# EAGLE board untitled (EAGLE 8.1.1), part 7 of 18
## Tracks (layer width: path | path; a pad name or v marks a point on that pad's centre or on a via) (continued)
S$6634 (continued)
  Bottom 0: 111.83,160.68 111.78,160.73
S$6635
  Bottom 0: 111.78,160.73 111.71,160.77
S$6636
  Bottom 0: 111.71,160.77 111.63,160.78
S$6637
  Bottom 0: 111.63,160.78 111.19,160.78
S$6638
  Bottom 0: 111.19,160.78 111.19,160.91
S$6639
  Bottom 0: 111.19,160.91 111.12,161.13
S$6640
  Bottom 0: 111.12,161.13 110.96,161.29
S$6641
  Bottom 0: 110.96,161.29 110.74,161.35
S$6642
  Bottom 0: 110.74,161.35 110.39,161.35
S$6643
  Bottom 0: 110.39,161.35 109.3,162.43
S$6644
  Bottom 0: 109.3,162.43 109.36,162.57
S$6645
  Bottom 0: 109.36,162.57 109.41,162.89
S$6646
  Bottom 0: 109.41,162.89 109.36,163.22
S$6647
  Bottom 0: 109.36,163.22 109.23,163.51
S$6648
  Bottom 0: 109.23,163.51 109.03,163.77
S$6649
  Bottom 0: 109.03,163.77 108.76,163.96
S$6650
  Bottom 0: 108.76,163.96 108.46,164.06
S$6651
  Bottom 0: 108.46,164.06 108.13,164.08
S$6652
  Bottom 0: 108.13,164.08 107.81,164.02
S$6653
  Bottom 0: 107.81,164.02 107.52,163.87
S$6654
  Bottom 0: 107.52,163.87 107.29,163.65
S$6655
  Bottom 0: 107.29,163.65 107.12,163.37
S$6656
  Bottom 0: 107.12,163.37 107.03,163.06
S$6657
  Bottom 0: 107.03,163.06 107.03,162.73
S$6658
  Bottom 0: 107.03,162.73 107.12,162.42
S$6659
  Bottom 0: 107.12,162.42 107.29,162.14
S$6660
  Bottom 0: 107.29,162.14 107.52,161.92
S$6661
  Bottom 0: 107.52,161.92 107.81,161.77
S$6662
  Bottom 0: 107.81,161.77 108.13,161.71
S$6663
  Bottom 0: 108.13,161.71 108.46,161.73
S$6664
  Bottom 0: 108.46,161.73 108.68,161.8
S$6665
  Bottom 0: 108.68,161.8 109.74,160.75
S$6666
  Bottom 0: 109.74,160.75 109.7,160.73
S$6667
  Bottom 0: 109.7,160.73 109.65,160.68
S$6668
  Bottom 0: 109.65,160.68 109.61,160.6
S$6669
  Bottom 0: 109.61,160.6 109.6,160.53
S$6670
  Bottom 0: 109.6,160.53 109.6,159.04
S$6671
  Bottom 0: 109.6,159.04 105.97,162.67
S$6672
  Bottom 0: 105.97,162.67 106.01,162.88
S$6673
  Bottom 0: 106.01,162.88 105.96,163.13
S$6674
  Bottom 0: 105.96,163.13 105.83,163.34
S$6675
  Bottom 0: 105.83,163.34 105.63,163.5
S$6676
  Bottom 0: 105.63,163.5 105.4,163.55
S$6677
  Bottom 0: 105.4,163.55 105.97,164.13
S$6678
  Bottom 0: 105.97,164.13 106.23,164.08
S$6679
  Bottom 0: 106.23,164.08 106.55,164.1
S$6680
  Bottom 0: 106.55,164.1 106.86,164.21
S$6681
  Bottom 0: 106.86,164.21 107.12,164.39
S$6682
  Bottom 0: 107.12,164.39 107.33,164.65
S$6683
  Bottom 0: 107.33,164.65 107.45,164.95
S$6684
  Bottom 0: 107.45,164.95 107.5,165.27
S$6685
  Bottom 0: 107.5,165.27 107.45,165.59
S$6686
  Bottom 0: 107.45,165.59 107.33,165.89
S$6687
  Bottom 0: 107.33,165.89 107.12,166.14
S$6688
  Bottom 0: 107.12,166.14 107.98,166.14
S$6689
  Bottom 0: 107.98,166.14 113.35,160.77
S$6690
  Bottom 0: 113.35,160.77 113.12,160.77
S$6691
  Bottom 0: 113.12,160.77 112.81,160.68
S$6692
  Bottom 0: 112.81,160.68 112.53,160.5
S$6693
  Bottom 0: 112.53,160.5 112.32,160.26
S$6694
  Bottom 0: 112.32,160.26 112.18,159.96
S$6695
  Bottom 0: 112.18,159.96 112.14,159.64
S$6696
  Bottom 0: 112.14,159.64 112.18,159.32
S$6697
  Bottom 0: 112.18,159.32 112.32,159.02
S$6698
  Bottom 0: 112.32,159.02 112.53,158.78
S$6699
  Bottom 0: 112.53,158.78 112.81,158.6
S$6700
  Bottom 0: 112.81,158.6 113.12,158.51
S$6701
  Bottom 0: 113.12,158.51 113.45,158.51
S$6702
  Bottom 0: 113.45,158.51 113.76,158.6
S$6703
  Bottom 0: 113.76,158.6 114.03,158.78
S$6704
  Bottom 0: 114.03,158.78 114.24,159.02
S$6705
  Bottom 0: 114.24,159.02 114.38,159.32
S$6706
  Bottom 0: 114.38,159.32 114.43,159.64
S$6707
  Bottom 0: 114.43,159.64 114.42,159.71
S$6708
  Bottom 0: 114.42,159.71 123.49,150.63
S$6709
  Bottom 0: 123.49,150.63 123.49,131.46
S$6710
  Bottom 0: 123.49,131.46 113.33,121.3
S$6711
  Bottom 0: 113.33,121.3 113.29,121.24
S$6712
  Bottom 0: 113.29,121.24 113.25,121.18
S$6713
  Bottom 0: 113.25,121.18 113.22,121.12
S$6714
  Bottom 0: 113.22,121.12 113.21,121.06
S$6715
  Bottom 0: 113.21,121.06 113.2,120.98
S$6716
  Bottom 0: 113.2,120.98 113.2,113.26
S$6717
  Bottom 0: 113.2,113.26 113.06,113.11
S$6718
  Bottom 0: 113.06,113.11 112.97,112.88
S$6719
  Bottom 0: 112.97,112.88 112.97,112.62
S$6720
  Bottom 0: 112.97,112.62 113.06,112.39
S$6721
  Bottom 0: 113.06,112.39 113.23,112.2
S$6722
  Bottom 0: 113.23,112.2 113.45,112.09
S$6723
  Bottom 0: 113.45,112.09 113.71,112.07
S$6724
  Bottom 0: 113.71,112.07 113.95,112.14
S$6725
  Bottom 0: 113.95,112.14 114.15,112.29
S$6726
  Bottom 0: 114.15,112.29 114.28,112.5
S$6727
  Bottom 0: 114.28,112.5 114.33,112.75
S$6728
  Bottom 0: 114.33,112.75 114.28,113
S$6729
  Bottom 0: 114.28,113 114.15,113.21
S$6730
  Bottom 0: 114.15,113.21 114.09,113.26
S$6731
  Bottom 0: 114.09,113.26 114.09,120.8
S$6732
  Bottom 0: 114.09,120.8 124.25,130.96
S$6733
  Bottom 0: 124.25,130.96 124.29,131.01
S$6734
  Bottom 0: 124.29,131.01 124.33,131.07
S$6735
  Bottom 0: 124.33,131.07 124.35,131.13
S$6736
  Bottom 0: 124.35,131.13 124.37,131.2
S$6737
  Bottom 0: 124.37,131.2 124.37,131.27
S$6738
  Bottom 0: 124.37,131.27 124.37,147.41
S$6739
  Bottom 0: 124.37,147.41 130.71,147.41
S$6740
  Bottom 0: 130.71,147.41 130.78,147.42
S$6741
  Bottom 0: 130.78,147.42 130.85,147.43
S$6742
  Bottom 0: 130.85,147.43 130.91,147.46
S$6743
  Bottom 0: 130.91,147.46 130.97,147.5
S$6744
  Bottom 0: 130.97,147.5 131.02,147.54
S$6745
  Bottom 0: 131.02,147.54 134.25,150.77
S$6746
  Bottom 0: 134.25,150.77 134.28,150.75
S$6747
  Bottom 0: 134.28,150.75 134.61,150.65
S$6748
  Bottom 0: 134.61,150.65 134.96,150.63
S$6749
  Bottom 0: 134.96,150.63 135.31,150.69
S$6750
  Bottom 0: 135.31,150.69 135.62,150.84
S$6751
  Bottom 0: 135.62,150.84 135.89,151.06
S$6752
  Bottom 0: 135.89,151.06 136.1,151.35
S$6753
  Bottom 0: 136.1,151.35 136.22,151.67
S$6754
  Bottom 0: 136.22,151.67 136.27,152.02
S$6755
  Bottom 0: 136.27,152.02 136.22,152.36
S$6756
  Bottom 0: 136.22,152.36 136.1,152.69
S$6757
  Bottom 0: 136.1,152.69 135.89,152.97
S$6758
  Bottom 0: 135.89,152.97 135.62,153.2
S$6759
  Bottom 0: 135.62,153.2 135.31,153.35
S$6760
  Bottom 0: 135.31,153.35 134.96,153.41
S$6761
  Bottom 0: 134.96,153.41 134.61,153.39
S$6762
  Bottom 0: 134.61,153.39 134.28,153.28
S$6763
  Bottom 0: 134.28,153.28 133.99,153.1
S$6764
  Bottom 0: 133.99,153.1 133.74,152.84
S$6765
  Bottom 0: 133.74,152.84 133.57,152.53
S$6766
  Bottom 0: 133.57,152.53 133.49,152.19
S$6767
  Bottom 0: 133.49,152.19 133.49,151.84
S$6768
  Bottom 0: 133.49,151.84 133.57,151.51
S$6769
  Bottom 0: 133.57,151.51 133.63,151.4
S$6770
  Bottom 0: 133.63,151.4 130.52,148.29
S$6771
  Bottom 0: 130.52,148.29 129.26,148.29
S$6772
  Bottom 0: 129.26,148.29 129.27,148.3
S$6773
  Bottom 0: 129.27,148.3 129.54,148.52
S$6774
  Bottom 0: 129.54,148.52 129.75,148.81
S$6775
  Bottom 0: 129.75,148.81 129.88,149.13
S$6776
  Bottom 0: 129.88,149.13 129.92,149.48
S$6777
  Bottom 0: 129.92,149.48 129.88,149.82
S$6778
  Bottom 0: 129.88,149.82 129.75,150.15
S$6779
  Bottom 0: 129.75,150.15 129.54,150.43
S$6780
  Bottom 0: 129.54,150.43 129.27,150.66
S$6781
  Bottom 0: 129.27,150.66 128.96,150.81
S$6782
  Bottom 0: 128.96,150.81 128.61,150.87
S$6783
  Bottom 0: 128.61,150.87 128.26,150.85
S$6784
  Bottom 0: 128.26,150.85 127.93,150.74
S$6785
  Bottom 0: 127.93,150.74 127.64,150.56
S$6786
  Bottom 0: 127.64,150.56 127.39,150.3
S$6787
  Bottom 0: 127.39,150.3 127.22,149.99
S$6788
  Bottom 0: 127.22,149.99 127.14,149.65
S$6789
  Bottom 0: 127.14,149.65 127.14,149.3
S$6790
  Bottom 0: 127.14,149.3 127.22,148.97
S$6791
  Bottom 0: 127.22,148.97 127.39,148.66
S$6792
  Bottom 0: 127.39,148.66 127.64,148.4
S$6793
  Bottom 0: 127.64,148.4 127.8,148.29
S$6794
  Bottom 0: 127.8,148.29 124.37,148.29
S$6795
  Bottom 0: 124.37,148.29 124.37,150.81
S$6796
  Bottom 0: 124.37,150.81 124.37,150.89
S$6797
  Bottom 0: 124.37,150.89 124.35,150.95
S$6798
  Bottom 0: 124.35,150.95 124.33,151.01
S$6799
  Bottom 0: 124.33,151.01 124.29,151.07
S$6800
  Bottom 0: 124.29,151.07 124.25,151.13
S$6801
  Bottom 0: 124.25,151.13 108.48,166.9
S$6802
  Bottom 0: 108.48,166.9 108.37,166.98
S$6803
  Bottom 0: 108.37,166.98 108.31,167
S$6804
  Bottom 0: 108.31,167 108.24,167.02
S$6805
  Bottom 0: 108.24,167.02 108.17,167.03
S$6806
  Bottom 0: 108.17,167.03 104.53,167.03
S$6807
  Bottom 0: 104.53,167.03 104.45,167.02
S$6808
  Bottom 0: 104.45,167.02 104.39,167
S$6809
  Bottom 0: 104.39,167 104.32,166.97
S$6810
  Bottom 0: 104.32,166.97 104.27,166.94
S$6811
  Bottom 0: 104.27,166.94 104.21,166.89
S$6812
  Bottom 0: 104.21,166.89 101.72,164.4
S$6813
  Bottom 0: 101.72,164.4 99.51,164.4
S$6814
  Bottom 0: 99.51,164.4 99.71,164.65
S$6815
  Bottom 0: 99.71,164.65 99.83,164.95
S$6816
  Bottom 0: 99.83,164.95 99.88,165.27
S$6817
  Bottom 0: 99.88,165.27 99.83,165.59
S$6818
  Bottom 0: 99.83,165.59 99.71,165.89
S$6819
  Bottom 0: 99.71,165.89 99.5,166.14
S$6820
  Bottom 0: 99.5,166.14 99.24,166.33
S$6821
  Bottom 0: 99.24,166.33 98.93,166.44
S$6822
  Bottom 0: 98.93,166.44 98.63,166.46
S$6823
  Bottom 0: 98.63,166.46 98.63,168.08
S$6824
  Bottom 0: 98.63,168.08 98.65,168.02
S$6825
  Bottom 0: 98.65,168.02 98.82,167.71
S$6826
  Bottom 0: 98.82,167.71 99.06,167.45
S$6827
  Bottom 0: 99.06,167.45 99.36,167.26
S$6828
  Bottom 0: 99.36,167.26 99.69,167.16
S$6829
  Bottom 0: 99.69,167.16 100.03,167.14
S$6830
  Bottom 0: 100.03,167.14 100.38,167.2
S$6831
  Bottom 0: 100.38,167.2 100.7,167.35
S$6832
  Bottom 0: 100.7,167.35 100.97,167.57
S$6833
  Bottom 0: 100.97,167.57 101.17,167.86
S$6834
  Bottom 0: 101.17,167.86 101.3,168.18
S$6835
  Bottom 0: 101.3,168.18 101.35,168.53
S$6836
  Bottom 0: 101.35,168.53 101.3,168.87
S$6837
  Bottom 0: 101.3,168.87 101.17,169.2
S$6838
  Bottom 0: 101.17,169.2 100.97,169.48
S$6839
  Bottom 0: 100.97,169.48 100.7,169.71
S$6840
  Bottom 0: 100.7,169.71 100.38,169.86
S$6841
  Bottom 0: 100.38,169.86 100.03,169.92
S$6842
  Bottom 0: 100.03,169.92 99.69,169.9
S$6843
  Bottom 0: 99.69,169.9 99.36,169.79
S$6844
  Bottom 0: 99.36,169.79 99.06,169.61
S$6845
  Bottom 0: 99.06,169.61 98.82,169.35
S$6846
  Bottom 0: 98.82,169.35 98.65,169.04
S$6847
  Bottom 0: 98.65,169.04 98.63,168.99
S$6848
  Bottom 0: 98.63,168.99 98.63,174.21
S$6849
  Bottom 0: 98.63,174.21 101.53,177.1
S$6850
  Bottom 0: 101.53,177.1 101.56,177.16
S$6851
  Bottom 0: 101.56,177.16 101.6,177.2
S$6852
  Bottom 0: 101.6,177.2 101.61,177.25
S$6853
  Bottom 0: 101.61,177.25 101.64,177.3
S$6854
  Bottom 0: 101.64,177.3 101.64,177.36
S$6855
  Bottom 0: 101.64,177.36 101.66,177.42
S$6856
  Bottom 0: 101.66,177.42 101.66,177.55
S$6857
  Bottom 0: 101.66,177.55 102.11,177.55
S$6858
  Bottom 0: 102.11,177.55 102.18,177.56
S$6859
  Bottom 0: 102.18,177.56 102.25,177.6
S$6860
  Bottom 0: 102.25,177.6 102.31,177.65
S$6861
  Bottom 0: 102.31,177.65 102.35,177.72
S$6862
  Bottom 0: 102.35,177.72 102.36,177.8
S$6863
  Bottom 0: 102.36,177.8 102.36,179.51
S$6864
  Bottom 0: 102.36,179.51 102.97,179.51
S$6865
  Bottom 0: 102.97,179.51 102.8,179.31
S$6866
  Bottom 0: 102.8,179.31 102.66,179.01
S$6867
  Bottom 0: 102.66,179.01 102.62,178.69
S$6868
  Bottom 0: 102.62,178.69 102.66,178.37
S$6869
  Bottom 0: 102.66,178.37 102.8,178.07
S$6870
  Bottom 0: 102.8,178.07 103.01,177.82
S$6871
  Bottom 0: 103.01,177.82 103.29,177.65
S$6872
  Bottom 0: 103.29,177.65 103.6,177.56
S$6873
  Bottom 0: 103.6,177.56 103.92,177.56
S$6874
  Bottom 0: 103.92,177.56 104.23,177.65
S$6875
  Bottom 0: 104.23,177.65 104.51,177.82
S$6876
  Bottom 0: 104.51,177.82 104.72,178.07
S$6877
  Bottom 0: 104.72,178.07 104.86,178.37
S$6878
  Bottom 0: 104.86,178.37 104.9,178.69
S$6879
  Bottom 0: 104.9,178.69 104.86,179.01
S$6880
  Bottom 0: 104.86,179.01 104.72,179.31
S$6881
  Bottom 0: 104.72,179.31 104.55,179.51
S$6882
  Bottom 0: 104.55,179.51 119.13,179.51
S$6883
  Bottom 0: 119.13,179.51 119.13,177.8
S$6884
  Bottom 0: 119.13,177.8 119.14,177.72
S$6885
  Bottom 0: 119.14,177.72 119.18,177.65
S$6886
  Bottom 0: 119.18,177.65 119.23,177.6
S$6887
  Bottom 0: 119.23,177.6 119.3,177.56
S$6888
  Bottom 0: 119.3,177.56 119.38,177.55
S$6889
  Bottom 0: 119.38,177.55 119.77,177.55
S$6890
  Bottom 0: 119.77,177.55 117.11,174.89
S$6891
  Bottom 0: 117.11,174.89 117.07,174.84
S$6892
  Bottom 0: 117.07,174.84 117.03,174.78
S$6893
  Bottom 0: 117.03,174.78 117,174.72
S$6894
  Bottom 0: 117,174.72 116.99,174.65
S$6895
  Bottom 0: 116.99,174.65 116.98,174.58
S$6896
  Bottom 0: 116.98,174.58 116.98,166.19
S$6897
  Bottom 0: 116.98,166.19 116.81,166.03
S$6898
  Bottom 0: 116.81,166.03 116.64,165.75
S$6899
  Bottom 0: 116.64,165.75 116.56,165.43
S$6900
  Bottom 0: 116.56,165.43 116.56,165.11
S$6901
  Bottom 0: 116.56,165.11 116.64,164.79
S$6902
  Bottom 0: 116.64,164.79 116.71,164.68
S$6903
  Bottom 0: 116.71,164.68 113.93,167.46
S$6904
  Bottom 0: 113.93,167.46 113.88,167.5
S$6905
  Bottom 0: 113.88,167.5 113.82,167.54
S$6906
  Bottom 0: 113.82,167.54 113.76,167.56
S$6907
  Bottom 0: 113.76,167.56 113.69,167.58
S$6908
  Bottom 0: 113.69,167.58 113.62,167.58
S$6909
  Bottom 0: 113.62,167.58 110.41,167.58
S$6910
  Bottom 0: 110.41,167.58 107.54,170.45
S$6911
  Bottom 0: 107.54,170.45 107.65,170.72
S$6912
  Bottom 0: 107.65,170.72 107.7,171.07
S$6913
  Bottom 0: 107.7,171.07 107.65,171.41
S$6914
  Bottom 0: 107.65,171.41 107.52,171.74
S$6915
  Bottom 0: 107.52,171.74 107.31,172.02
S$6916
  Bottom 0: 107.31,172.02 107.05,172.25
S$6917
  Bottom 0: 107.05,172.25 106.73,172.4
S$6918
  Bottom 0: 106.73,172.4 106.39,172.46
S$6919
  Bottom 0: 106.39,172.46 106.03,172.44
S$6920
  Bottom 0: 106.03,172.44 105.7,172.33
S$6921
  Bottom 0: 105.7,172.33 105.41,172.15
S$6922
  Bottom 0: 105.41,172.15 105.17,171.89
S$6923
  Bottom 0: 105.17,171.89 105,171.58
S$6924
  Bottom 0: 105,171.58 104.91,171.24
S$6925
  Bottom 0: 104.91,171.24 104.91,170.9
S$6926
  Bottom 0: 104.91,170.9 105,170.56
S$6927
  Bottom 0: 105,170.56 105.17,170.25
S$6928
  Bottom 0: 105.17,170.25 105.41,169.99
S$6929
  Bottom 0: 105.41,169.99 105.7,169.8
S$6930
  Bottom 0: 105.7,169.8 106.03,169.7
S$6931
  Bottom 0: 106.03,169.7 106.39,169.68
S$6932
  Bottom 0: 106.39,169.68 106.73,169.74
S$6933
  Bottom 0: 106.73,169.74 106.91,169.82
S$6934
  Bottom 0: 106.91,169.82 109.91,166.83
S$6935
  Bottom 0: 109.91,166.83 109.97,166.79
S$6936
  Bottom 0: 109.97,166.79 110.03,166.75
S$6937
  Bottom 0: 110.03,166.75 110.09,166.72
S$6938
  Bottom 0: 110.09,166.72 110.15,166.71
S$6939
  Bottom 0: 110.15,166.71 110.23,166.7
S$6940
  Bottom 0: 110.23,166.7 113.43,166.7
S$6941
  Bottom 0: 113.43,166.7 116.07,164.06
S$6942
  Bottom 0: 116.07,164.06 115.75,164.08
S$6943
  Bottom 0: 115.75,164.08 115.43,164.02
S$6944
  Bottom 0: 115.43,164.02 115.14,163.87
S$6945
  Bottom 0: 115.14,163.87 114.91,163.65
S$6946
  Bottom 0: 114.91,163.65 114.74,163.37
S$6947
  Bottom 0: 114.74,163.37 114.65,163.06
S$6948
  Bottom 0: 114.65,163.06 114.65,162.73
S$6949
  Bottom 0: 114.65,162.73 114.74,162.42
S$6950
  Bottom 0: 114.74,162.42 114.91,162.14
S$6951
  Bottom 0: 114.91,162.14 115.14,161.92
S$6952
  Bottom 0: 115.14,161.92 115.43,161.77
S$6953
  Bottom 0: 115.43,161.77 115.75,161.71
S$6954
  Bottom 0: 115.75,161.71 116.08,161.73
S$6955
  Bottom 0: 116.08,161.73 116.38,161.83
S$6956
  Bottom 0: 116.38,161.83 116.65,162.02
S$6957
  Bottom 0: 116.65,162.02 116.85,162.28
S$6958
  Bottom 0: 116.85,162.28 116.88,162.33
S$6959
  Bottom 0: 116.88,162.33 123.05,162.33
S$6960
  Bottom 0: 123.05,162.33 123.14,162.33
S$6961
  Bottom 0: 123.14,162.33 123.23,162.35
S$6962
  Bottom 0: 123.23,162.35 123.31,162.38
S$6963
  Bottom 0: 123.31,162.38 123.38,162.43
S$6964
  Bottom 0: 123.38,162.43 123.45,162.49
S$6965
  Bottom 0: 123.45,162.49 125.08,164.12
S$6966
  Bottom 0: 125.08,164.12 125.28,164.08
S$6967
  Bottom 0: 125.28,164.08 125.6,164.1
S$6968
  Bottom 0: 125.6,164.1 125.91,164.21
S$6969
  Bottom 0: 125.91,164.21 126.17,164.4
S$6970
  Bottom 0: 126.17,164.4 126.37,164.64
S$6971
  Bottom 0: 126.37,164.64 132.34,164.64
S$6972
  Bottom 0: 132.34,164.64 133.75,163.23
S$6973
  Bottom 0: 133.75,163.23 133.71,163.06
S$6974
  Bottom 0: 133.71,163.06 133.71,162.73
S$6975
  Bottom 0: 133.71,162.73 133.79,162.42
S$6976
  Bottom 0: 133.79,162.42 133.96,162.14
S$6977
  Bottom 0: 133.96,162.14 134.2,161.92
S$6978
  Bottom 0: 134.2,161.92 134.49,161.77
S$6979
  Bottom 0: 134.49,161.77 134.81,161.71
S$6980
  Bottom 0: 134.81,161.71 135.13,161.73
S$6981
  Bottom 0: 135.13,161.73 135.44,161.83
S$6982
  Bottom 0: 135.44,161.83 135.7,162.02
S$6983
  Bottom 0: 135.7,162.02 135.91,162.28
S$6984
  Bottom 0: 135.91,162.28 136.04,162.57
S$6985
  Bottom 0: 136.04,162.57 136.08,162.89
S$6986
  Bottom 0: 136.08,162.89 136.04,163.22
S$6987
  Bottom 0: 136.04,163.22 135.96,163.39
S$6988
  Bottom 0: 135.96,163.39 145.01,163.39
S$6989
  Bottom 0: 145.01,163.39 145.08,163.4
S$6990
  Bottom 0: 145.08,163.4 145.15,163.41
S$6991
  Bottom 0: 145.15,163.41 145.2,163.44
S$6992
  Bottom 0: 145.2,163.44 145.26,163.48
S$6993
  Bottom 0: 145.26,163.48 145.31,163.51
S$6994
  Bottom 0: 145.31,163.51 145.22,163.37
S$6995
  Bottom 0: 145.22,163.37 145.14,163.06
S$6996
  Bottom 0: 145.14,163.06 145.14,162.73
S$6997
  Bottom 0: 145.14,162.73 145.22,162.42
S$6998
  Bottom 0: 145.22,162.42 145.39,162.14
S$6999
  Bottom 0: 145.39,162.14 145.63,161.92
S$7000
  Bottom 0: 145.63,161.92 145.92,161.77
S$7001
  Bottom 0: 145.92,161.77 146.24,161.71
S$7002
  Bottom 0: 146.24,161.71 146.56,161.73
S$7003
  Bottom 0: 146.56,161.73 146.78,161.8
S$7004
  Bottom 0: 146.78,161.8 147.84,160.75
S$7005
  Bottom 0: 147.84,160.75 147.81,160.73
S$7006
  Bottom 0: 147.81,160.73 147.75,160.68
S$7007
  Bottom 0: 147.75,160.68 147.71,160.6
S$7008
  Bottom 0: 147.71,160.6 147.7,160.53
S$7009
  Bottom 0: 147.7,160.53 147.7,158.75
S$7010
  Bottom 0: 147.7,158.75 147.71,158.67
S$7011
  Bottom 0: 147.71,158.67 147.75,158.6
S$7012
  Bottom 0: 147.75,158.6 147.81,158.55
S$7013
  Bottom 0: 147.81,158.55 147.88,158.51
S$7014
  Bottom 0: 147.88,158.51 147.96,158.5
S$7015
  Bottom 0: 147.96,158.5 149.44,158.5
S$7016
  Bottom 0: 149.44,158.5 146.36,155.42
S$7017
  Bottom 0: 146.36,155.42 141.47,160.31
S$7018
  Bottom 0: 141.47,160.31 141.4,160.37
S$7019
  Bottom 0: 141.4,160.37 141.33,160.41
S$7020
  Bottom 0: 141.33,160.41 141.24,160.45
S$7021
  Bottom 0: 141.24,160.45 141.16,160.47
S$7022
  Bottom 0: 141.16,160.47 141.07,160.47
S$7023
  Bottom 0: 141.07,160.47 133.1,160.47
S$7024
  Bottom 0: 133.1,160.47 133.08,160.5
S$7025
  Bottom 0: 133.08,160.5 132.81,160.68
S$7026
  Bottom 0: 132.81,160.68 132.5,160.77
S$7027
  Bottom 0: 132.5,160.77 132.17,160.77
S$7028
  Bottom 0: 132.17,160.77 131.86,160.68
S$7029
  Bottom 0: 131.86,160.68 131.59,160.5
S$7030
  Bottom 0: 131.59,160.5 131.37,160.26
S$7031
  Bottom 0: 131.37,160.26 131.23,159.96
S$7032
  Bottom 0: 131.23,159.96 131.19,159.64
S$7033
  Bottom 0: 131.19,159.64 131.23,159.32
S$7034
  Bottom 0: 131.23,159.32 131.37,159.02
S$7035
  Bottom 0: 131.37,159.02 131.59,158.78
S$7036
  Bottom 0: 131.59,158.78 131.7,158.7
S$7037
  Bottom 0: 131.7,158.7 130.93,158.7
S$7038
  Bottom 0: 130.93,158.7 130.94,158.75
S$7039
  Bottom 0: 130.94,158.75 130.94,160.53
S$7040
  Bottom 0: 130.94,160.53 130.93,160.6
S$7041
  Bottom 0: 130.93,160.6 130.88,160.68
S$7042
  Bottom 0: 130.88,160.68 130.83,160.73
S$7043
  Bottom 0: 130.83,160.73 130.76,160.77
S$7044
  Bottom 0: 130.76,160.77 130.68,160.78
S$7045
  Bottom 0: 130.68,160.78 130.24,160.78
S$7046
  Bottom 0: 130.24,160.78 130.24,160.91
S$7047
  Bottom 0: 130.24,160.91 130.18,161.13
S$7048
  Bottom 0: 130.18,161.13 130.01,161.29
S$7049
  Bottom 0: 130.01,161.29 129.79,161.35
S$7050
  Bottom 0: 129.79,161.35 129.44,161.35
S$7051
  Bottom 0: 129.44,161.35 128.36,162.44
S$7052
  Bottom 0: 128.36,162.44 128.42,162.57
S$7053
  Bottom 0: 128.42,162.57 128.46,162.89
S$7054
  Bottom 0: 128.46,162.89 128.42,163.22
S$7055
  Bottom 0: 128.42,163.22 128.29,163.51
S$7056
  Bottom 0: 128.29,163.51 128.08,163.77
S$7057
  Bottom 0: 128.08,163.77 127.82,163.96
S$7058
  Bottom 0: 127.82,163.96 127.51,164.06
S$7059
  Bottom 0: 127.51,164.06 127.19,164.08
S$7060
  Bottom 0: 127.19,164.08 126.87,164.02
S$7061
  Bottom 0: 126.87,164.02 126.58,163.87
S$7062
  Bottom 0: 126.58,163.87 126.34,163.65
S$7063
  Bottom 0: 126.34,163.65 126.17,163.37
S$7064
  Bottom 0: 126.17,163.37 126.09,163.06
S$7065
  Bottom 0: 126.09,163.06 126.09,162.73
S$7066
  Bottom 0: 126.09,162.73 126.17,162.42
S$7067
  Bottom 0: 126.17,162.42 126.34,162.14
S$7068
  Bottom 0: 126.34,162.14 126.58,161.92
S$7069
  Bottom 0: 126.58,161.92 126.87,161.77
S$7070
  Bottom 0: 126.87,161.77 127.19,161.71
S$7071
  Bottom 0: 127.19,161.71 127.51,161.73
S$7072
  Bottom 0: 127.51,161.73 127.73,161.8
S$7073
  Bottom 0: 127.73,161.8 128.79,160.75
S$7074
  Bottom 0: 128.79,160.75 128.75,160.73
S$7075
  Bottom 0: 128.75,160.73 128.7,160.68
S$7076
  Bottom 0: 128.7,160.68 128.66,160.6
S$7077
  Bottom 0: 128.66,160.6 128.65,160.53
S$7078
  Bottom 0: 128.65,160.53 128.65,158.75
S$7079
  Bottom 0: 128.65,158.75 128.66,158.7
S$7080
  Bottom 0: 128.66,158.7 122.55,158.7
S$7081
  Bottom 0: 122.55,158.7 122.52,158.9
S$7082
  Bottom 0: 122.52,158.9 122.39,159.18
S$7083
  Bottom 0: 122.39,159.18 122.18,159.4
S$7084
  Bottom 0: 122.18,159.4 121.92,159.55
S$7085
  Bottom 0: 121.92,159.55 121.62,159.61
S$7086
  Bottom 0: 121.62,159.61 121.32,159.59
S$7087
  Bottom 0: 121.32,159.59 121.04,159.48
S$7088
  Bottom 0: 121.04,159.48 120.8,159.29
S$7089
  Bottom 0: 120.8,159.29 120.64,159.04
S$7090
  Bottom 0: 120.64,159.04 120.54,158.75
S$7091
  Bottom 0: 120.54,158.75 120.54,158.45
S$7092
  Bottom 0: 120.54,158.45 120.64,158.16
S$7093
  Bottom 0: 120.64,158.16 120.8,157.91
S$7094
  Bottom 0: 120.8,157.91 121.04,157.72
S$7095
  Bottom 0: 121.04,157.72 121.32,157.61
S$7096
  Bottom 0: 121.32,157.61 121.62,157.59
S$7097
  Bottom 0: 121.62,157.59 121.92,157.66
S$7098
  Bottom 0: 121.92,157.66 122.18,157.81
S$7099
  Bottom 0: 122.18,157.81 122.19,157.82
S$7100
  Bottom 0: 122.19,157.82 139.96,157.82
S$7101
  Bottom 0: 139.96,157.82 140.09,157.72
S$7102
  Bottom 0: 140.09,157.72 140.37,157.61
S$7103
  Bottom 0: 140.37,157.61 140.67,157.59
S$7104
  Bottom 0: 140.67,157.59 140.97,157.66
S$7105
  Bottom 0: 140.97,157.66 141.23,157.81
S$7106
  Bottom 0: 141.23,157.81 141.43,158.03
S$7107
  Bottom 0: 141.43,158.03 141.56,158.3
S$7108
  Bottom 0: 141.56,158.3 141.6,158.57
S$7109
  Bottom 0: 141.6,158.57 145.56,154.62
S$7110
  Bottom 0: 145.56,154.62 141.51,150.57
S$7111
  Bottom 0: 141.51,150.57 141.56,150.68
S$7112
  Bottom 0: 141.56,150.68 141.61,150.98
S$7113
  Bottom 0: 141.61,150.98 141.56,151.28
S$7114
  Bottom 0: 141.56,151.28 141.43,151.56
S$7115
  Bottom 0: 141.43,151.56 141.23,151.78
S$7116
  Bottom 0: 141.23,151.78 140.97,151.93
S$7117
  Bottom 0: 140.97,151.93 140.67,151.99
S$7118
  Bottom 0: 140.67,151.99 140.37,151.97
S$7119
  Bottom 0: 140.37,151.97 140.09,151.86
S$7120
  Bottom 0: 140.09,151.86 139.85,151.67
S$7121
  Bottom 0: 139.85,151.67 139.68,151.43
S$7122
  Bottom 0: 139.68,151.43 139.59,151.13
S$7123
  Bottom 0: 139.59,151.13 139.59,150.83
S$7124
  Bottom 0: 139.59,150.83 139.68,150.54
S$7125
  Bottom 0: 139.68,150.54 139.85,150.29
S$7126
  Bottom 0: 139.85,150.29 140.09,150.1
S$7127
  Bottom 0: 140.09,150.1 140.37,149.99
S$7128
  Bottom 0: 140.37,149.99 140.67,149.97
S$7129
  Bottom 0: 140.67,149.97 140.97,150.04
S$7130
  Bottom 0: 140.97,150.04 141,150.05
S$7131
  Bottom 0: 141,150.05 136.69,145.75
S$7132
  Bottom 0: 136.69,145.75 136.63,145.68
S$7133
  Bottom 0: 136.63,145.68 136.59,145.61
S$7134
  Bottom 0: 136.59,145.61 136.55,145.53
S$7135
  Bottom 0: 136.55,145.53 136.53,145.44
S$7136
  Bottom 0: 136.53,145.44 136.53,145.35
S$7137
  Bottom 0: 136.53,145.35 136.53,141.57
S$7138
  Bottom 0: 136.53,141.57 136.34,141.45
S$7139
  Bottom 0: 136.34,141.45 136.13,141.21
S$7140
  Bottom 0: 136.13,141.21 135.99,140.91
S$7141
  Bottom 0: 135.99,140.91 135.95,140.59
S$7142
  Bottom 0: 135.95,140.59 135.99,140.27
S$7143
  Bottom 0: 135.99,140.27 136.13,139.97
S$7144
  Bottom 0: 136.13,139.97 136.34,139.74
S$7145
  Bottom 0: 136.34,139.74 135.7,139.74
S$7146
  Bottom 0: 135.7,139.74 135.7,141.48
S$7147
  Bottom 0: 135.7,141.48 135.69,141.55
S$7148
  Bottom 0: 135.69,141.55 135.65,141.62
S$7149
  Bottom 0: 135.65,141.62 135.59,141.68
S$7150
  Bottom 0: 135.59,141.68 135.52,141.72
S$7151
  Bottom 0: 135.52,141.72 135.44,141.73
S$7152
  Bottom 0: 135.44,141.73 135,141.73
S$7153
  Bottom 0: 135,141.73 135,141.86
S$7154
  Bottom 0: 135,141.86 134.94,142.08
S$7155
  Bottom 0: 134.94,142.08 134.77,142.24
S$7156
  Bottom 0: 134.77,142.24 134.55,142.3
S$7157
  Bottom 0: 134.55,142.3 134.2,142.3
S$7158
  Bottom 0: 134.2,142.3 133.12,143.39
S$7159
  Bottom 0: 133.12,143.39 133.18,143.52
S$7160
  Bottom 0: 133.18,143.52 133.22,143.84
S$7161
  Bottom 0: 133.22,143.84 133.18,144.16
S$7162
  Bottom 0: 133.18,144.16 133.05,144.47
S$7163
  Bottom 0: 133.05,144.47 132.84,144.72
S$7164
  Bottom 0: 132.84,144.72 132.58,144.91
S$7165
  Bottom 0: 132.58,144.91 132.27,145.01
S$7166
  Bottom 0: 132.27,145.01 131.95,145.03
S$7167
  Bottom 0: 131.95,145.03 131.63,144.97
S$7168
  Bottom 0: 131.63,144.97 131.34,144.82
S$7169
  Bottom 0: 131.34,144.82 131.1,144.6
S$7170
  Bottom 0: 131.1,144.6 130.93,144.32
S$7171
  Bottom 0: 130.93,144.32 130.85,144.01
S$7172
  Bottom 0: 130.85,144.01 130.85,143.68
S$7173
  Bottom 0: 130.85,143.68 130.93,143.37
S$7174
  Bottom 0: 130.93,143.37 131.1,143.09
S$7175
  Bottom 0: 131.1,143.09 131.34,142.87
S$7176
  Bottom 0: 131.34,142.87 131.63,142.72
S$7177
  Bottom 0: 131.63,142.72 131.95,142.66
S$7178
  Bottom 0: 131.95,142.66 132.27,142.68
S$7179
  Bottom 0: 132.27,142.68 132.49,142.75
S$7180
  Bottom 0: 132.49,142.75 133.55,141.7
S$7181
  Bottom 0: 133.55,141.7 133.52,141.68
S$7182
  Bottom 0: 133.52,141.68 133.46,141.62
S$7183
  Bottom 0: 133.46,141.62 133.42,141.55
S$7184
  Bottom 0: 133.42,141.55 133.41,141.48
S$7185
  Bottom 0: 133.41,141.48 133.41,139.74
S$7186
  Bottom 0: 133.41,139.74 127.3,139.74
S$7187
  Bottom 0: 127.3,139.74 127.27,139.85
S$7188
  Bottom 0: 127.27,139.85 127.14,140.13
S$7189
  Bottom 0: 127.14,140.13 126.94,140.34
S$7190
  Bottom 0: 126.94,140.34 126.67,140.5
S$7191
  Bottom 0: 126.67,140.5 126.38,140.56
S$7192
  Bottom 0: 126.38,140.56 126.08,140.54
S$7193
  Bottom 0: 126.08,140.54 125.8,140.43
S$7194
  Bottom 0: 125.8,140.43 125.56,140.24
S$7195
  Bottom 0: 125.56,140.24 125.39,140
S$7196
  Bottom 0: 125.39,140 125.3,139.71
S$7197
  Bottom 0: 125.3,139.71 125.3,139.4
S$7198
  Bottom 0: 125.3,139.4 125.39,139.11
S$7199
  Bottom 0: 125.39,139.11 125.56,138.86
S$7200
  Bottom 0: 125.56,138.86 125.8,138.67
S$7201
  Bottom 0: 125.8,138.67 126.08,138.56
S$7202
  Bottom 0: 126.08,138.56 126.38,138.54
S$7203
  Bottom 0: 126.38,138.54 126.67,138.61
S$7204
  Bottom 0: 126.67,138.61 126.94,138.76
S$7205
  Bottom 0: 126.94,138.76 127.03,138.85
S$7206
  Bottom 0: 127.03,138.85 144.63,138.85
S$7207
  Bottom 0: 144.63,138.85 144.85,138.67
S$7208
  Bottom 0: 144.85,138.67 145.13,138.56
S$7209
  Bottom 0: 145.13,138.56 145.34,138.55
S$7210
  Bottom 0: 145.34,138.55 140.68,133.88
S$7211
  Bottom 0: 140.68,133.88 140.65,133.92
S$7212
  Bottom 0: 140.65,133.92 140.38,134.15
S$7213
  Bottom 0: 140.38,134.15 140.07,134.3
S$7214
  Bottom 0: 140.07,134.3 139.72,134.36
S$7215
  Bottom 0: 139.72,134.36 139.37,134.34
S$7216
  Bottom 0: 139.37,134.34 139.04,134.23
S$7217
  Bottom 0: 139.04,134.23 138.75,134.05
S$7218
  Bottom 0: 138.75,134.05 138.5,133.79
S$7219
  Bottom 0: 138.5,133.79 138.33,133.48
S$7220
  Bottom 0: 138.33,133.48 138.25,133.14
S$7221
  Bottom 0: 138.25,133.14 138.25,132.79
S$7222
  Bottom 0: 138.25,132.79 138.33,132.46
S$7223
  Bottom 0: 138.33,132.46 138.5,132.15
S$7224
  Bottom 0: 138.5,132.15 138.75,131.89
S$7225
  Bottom 0: 138.75,131.89 139.04,131.7
S$7226
  Bottom 0: 139.04,131.7 139.37,131.6
S$7227
  Bottom 0: 139.37,131.6 139.72,131.58
S$7228
  Bottom 0: 139.72,131.58 139.83,131.6
S$7229
  Bottom 0: 139.83,131.6 137.49,129.26
S$7230
  Bottom 0: 137.49,129.26 134.04,129.26
S$7231
  Bottom 0: 134.04,129.26 134.3,129.47
S$7232
  Bottom 0: 134.3,129.47 134.51,129.76
S$7233
  Bottom 0: 134.51,129.76 134.63,130.08
S$7234
  Bottom 0: 134.63,130.08 134.68,130.43
S$7235
  Bottom 0: 134.68,130.43 134.63,130.77
S$7236
  Bottom 0: 134.63,130.77 134.51,131.1
S$7237
  Bottom 0: 134.51,131.1 134.3,131.38
S$7238
  Bottom 0: 134.3,131.38 134.03,131.61
S$7239
  Bottom 0: 134.03,131.61 133.72,131.76
S$7240
  Bottom 0: 133.72,131.76 133.37,131.82
S$7241
  Bottom 0: 133.37,131.82 133.02,131.8
S$7242
  Bottom 0: 133.02,131.8 132.69,131.69
S$7243
  Bottom 0: 132.69,131.69 132.66,131.68
S$7244
  Bottom 0: 132.66,131.68 132.09,132.25
S$7245
  Bottom 0: 132.09,132.25 132.04,132.29
S$7246
  Bottom 0: 132.04,132.29 131.98,132.33
S$7247
  Bottom 0: 131.98,132.33 131.92,132.35
S$7248
  Bottom 0: 131.92,132.35 131.85,132.37
S$7249
  Bottom 0: 131.85,132.37 131.78,132.38
S$7250
  Bottom 0: 131.78,132.38 127.21,132.38
S$7251
  Bottom 0: 127.21,132.38 127.14,132.51
S$7252
  Bottom 0: 127.14,132.51 126.94,132.72
S$7253
  Bottom 0: 126.94,132.72 126.67,132.88
S$7254
  Bottom 0: 126.67,132.88 126.38,132.94
S$7255
  Bottom 0: 126.38,132.94 126.08,132.92
S$7256
  Bottom 0: 126.08,132.92 125.8,132.81
S$7257
  Bottom 0: 125.8,132.81 125.56,132.62
S$7258
  Bottom 0: 125.56,132.62 125.39,132.38
S$7259
  Bottom 0: 125.39,132.38 125.3,132.09
S$7260
  Bottom 0: 125.3,132.09 125.3,131.78
S$7261
  Bottom 0: 125.3,131.78 125.39,131.49
S$7262
  Bottom 0: 125.39,131.49 125.56,131.24
S$7263
  Bottom 0: 125.56,131.24 125.8,131.05
S$7264
  Bottom 0: 125.8,131.05 126.08,130.94
S$7265
  Bottom 0: 126.08,130.94 126.38,130.92
S$7266
  Bottom 0: 126.38,130.92 126.67,130.99
S$7267
  Bottom 0: 126.67,130.99 126.94,131.14
S$7268
  Bottom 0: 126.94,131.14 127.14,131.36
S$7269
  Bottom 0: 127.14,131.36 127.21,131.49
S$7270
  Bottom 0: 127.21,131.49 131.59,131.49
S$7271
  Bottom 0: 131.59,131.49 132.04,131.04
S$7272
  Bottom 0: 132.04,131.04 131.98,130.94
S$7273
  Bottom 0: 131.98,130.94 131.9,130.6
S$7274
  Bottom 0: 131.9,130.6 131.9,130.25
S$7275
  Bottom 0: 131.9,130.25 131.98,129.92
S$7276
  Bottom 0: 131.98,129.92 132.15,129.61
S$7277
  Bottom 0: 132.15,129.61 132.4,129.35
S$7278
  Bottom 0: 132.4,129.35 132.55,129.26
S$7279
  Bottom 0: 132.55,129.26 123.48,129.26
S$7280
  Bottom 0: 123.48,129.26 123.41,129.25
S$7281
  Bottom 0: 123.41,129.25 123.35,129.24
S$7282
  Bottom 0: 123.35,129.24 123.29,129.21
S$7283
  Bottom 0: 123.29,129.21 123.23,129.17
S$7284
  Bottom 0: 123.23,129.17 123.17,129.13
S$7285
  Bottom 0: 123.17,129.13 115.27,121.23
S$7286
  Bottom 0: 115.27,121.23 115.23,121.17
S$7287
  Bottom 0: 115.23,121.17 115.19,121.11
S$7288
  Bottom 0: 115.19,121.11 115.16,121.05
S$7289
  Bottom 0: 115.16,121.05 115.15,120.98
S$7290
  Bottom 0: 115.15,120.98 115.14,120.91
S$7291
  Bottom 0: 115.14,120.91 115.14,116.55
S$7292
  Bottom 0: 115.14,116.55 115.15,116.47
S$7293
  Bottom 0: 115.15,116.47 115.16,116.41
S$7294
  Bottom 0: 115.16,116.41 115.19,116.35
S$7295
  Bottom 0: 115.19,116.35 115.23,116.29
S$7296
  Bottom 0: 115.23,116.29 115.27,116.23
S$7297
  Bottom 0: 115.27,116.23 121.55,109.95
S$7298
  Bottom 0: 121.55,109.95 105.45,93.85
S$7299
  Bottom 0: 114,104.72 114.3,104.79
S$7300
  Bottom 0: 114.3,104.79 114.56,104.94
S$7301
  Bottom 0: 114.56,104.94 114.77,105.16
S$7302
  Bottom 0: 114.77,105.16 114.83,105.29
S$7303
  Bottom 0: 114.83,105.29 115.25,105.29
S$7304
  Bottom 0: 115.25,105.29 115.33,105.3
S$7305
  Bottom 0: 115.33,105.3 115.39,105.31
S$7306
  Bottom 0: 115.39,105.31 115.45,105.34
S$7307
  Bottom 0: 115.45,105.34 115.51,105.38
S$7308
  Bottom 0: 115.51,105.38 115.57,105.42
S$7309
  Bottom 0: 115.57,105.42 117.07,106.92
S$7310
  Bottom 0: 117.07,106.92 117.17,106.91
S$7311
  Bottom 0: 117.17,106.91 117.42,106.97
S$7312
  Bottom 0: 117.42,106.97 117.62,107.13
S$7313
  Bottom 0: 117.62,107.13 117.75,107.34
S$7314
  Bottom 0: 117.75,107.34 117.8,107.59
S$7315
  Bottom 0: 117.8,107.59 117.75,107.84
S$7316
  Bottom 0: 117.75,107.84 117.62,108.05
S$7317
  Bottom 0: 117.62,108.05 117.42,108.2
S$7318
  Bottom 0: 117.42,108.2 117.17,108.27
S$7319
  Bottom 0: 117.17,108.27 116.93,108.25
S$7320
  Bottom 0: 116.93,108.25 116.7,108.14
S$7321
  Bottom 0: 116.7,108.14 116.53,107.95
S$7322
  Bottom 0: 116.53,107.95 116.44,107.72
S$7323
  Bottom 0: 116.44,107.72 116.44,107.55
S$7324
  Bottom 0: 116.44,107.55 115.07,106.18
S$7325
  Bottom 0: 115.07,106.18 114.83,106.18
S$7326
  Bottom 0: 114.83,106.18 114.77,106.31
S$7327
  Bottom 0: 114.77,106.31 114.56,106.53
S$7328
  Bottom 0: 114.56,106.53 114.3,106.68
S$7329
  Bottom 0: 114.3,106.68 114,106.75
S$7330
  Bottom 0: 114,106.75 113.7,106.73
S$7331
  Bottom 0: 113.7,106.73 113.42,106.61
S$7332
  Bottom 0: 113.42,106.61 113.18,106.43
S$7333
  Bottom 0: 113.18,106.43 113.02,106.18
S$7334
  Bottom 0: 113.02,106.18 112.92,105.89
S$7335
  Bottom 0: 112.92,105.89 112.92,105.58
S$7336
  Bottom 0: 112.92,105.58 113.02,105.29
S$7337
  Bottom 0: 113.02,105.29 113.18,105.04
S$7338
  Bottom 0: 113.18,105.04 113.42,104.86
S$7339
  Bottom 0: 113.42,104.86 113.7,104.75
S$7340
  Bottom 0: 113.7,104.75 114,104.72
S$7341
  Bottom 0: 116.86,111.87 117.16,111.94
S$7342
  Bottom 0: 117.16,111.94 117.42,112.09
S$7343
  Bottom 0: 117.42,112.09 117.62,112.31
S$7344
  Bottom 0: 117.62,112.31 117.75,112.58
S$7345
  Bottom 0: 117.75,112.58 117.8,112.88
S$7346
  Bottom 0: 117.8,112.88 117.75,113.18
S$7347
  Bottom 0: 117.75,113.18 117.62,113.46
S$7348
  Bottom 0: 117.62,113.46 117.42,113.67
S$7349
  Bottom 0: 117.42,113.67 117.16,113.83
S$7350
  Bottom 0: 117.16,113.83 116.86,113.89
S$7351
  Bottom 0: 116.86,113.89 116.56,113.87
S$7352
  Bottom 0: 116.56,113.87 116.28,113.76
S$7353
  Bottom 0: 116.28,113.76 116.04,113.57
S$7354
  Bottom 0: 116.04,113.57 115.87,113.33
S$7355
  Bottom 0: 115.87,113.33 115.78,113.03
S$7356
  Bottom 0: 115.78,113.03 115.78,112.73
S$7357
  Bottom 0: 115.78,112.73 115.87,112.44
S$7358
  Bottom 0: 115.87,112.44 116.04,112.19
S$7359
  Bottom 0: 116.04,112.19 116.28,112
S$7360
  Bottom 0: 116.28,112 116.56,111.89
S$7361
  Bottom 0: 116.56,111.89 116.86,111.87
S$7362
  Bottom 0: 120.67,131.58 121.02,131.64
S$7363
  Bottom 0: 121.02,131.64 121.33,131.79
S$7364
  Bottom 0: 121.33,131.79 121.6,132.01
S$7365
  Bottom 0: 121.6,132.01 121.81,132.3
S$7366
  Bottom 0: 121.81,132.3 121.93,132.62
S$7367
  Bottom 0: 121.93,132.62 121.98,132.97
S$7368
  Bottom 0: 121.98,132.97 121.93,133.31
S$7369
  Bottom 0: 121.93,133.31 121.81,133.64
S$7370
  Bottom 0: 121.81,133.64 121.6,133.92
S$7371
  Bottom 0: 121.6,133.92 121.33,134.15
S$7372
  Bottom 0: 121.33,134.15 121.02,134.3
S$7373
  Bottom 0: 121.02,134.3 120.67,134.36
S$7374
  Bottom 0: 120.67,134.36 120.32,134.34
S$7375
  Bottom 0: 120.32,134.34 119.99,134.23
S$7376
  Bottom 0: 119.99,134.23 119.69,134.05
S$7377
  Bottom 0: 119.69,134.05 119.45,133.79
S$7378
  Bottom 0: 119.45,133.79 119.28,133.48
S$7379
  Bottom 0: 119.28,133.48 119.2,133.14
S$7380
  Bottom 0: 119.2,133.14 119.2,132.79
S$7381
  Bottom 0: 119.2,132.79 119.28,132.46
S$7382
  Bottom 0: 119.28,132.46 119.45,132.15
S$7383
  Bottom 0: 119.45,132.15 119.69,131.89
S$7384
  Bottom 0: 119.69,131.89 119.99,131.7
S$7385
  Bottom 0: 119.99,131.7 120.32,131.6
S$7386
  Bottom 0: 120.32,131.6 120.67,131.58
S$7387
  Bottom 0: 135.82,133.22 136.27,133.27
S$7388
  Bottom 0: 136.27,133.27 136.69,133.4
S$7389
  Bottom 0: 136.69,133.4 137.09,133.61
S$7390
  Bottom 0: 137.09,133.61 137.44,133.89
S$7391
  Bottom 0: 137.44,133.89 137.72,134.24
S$7392
  Bottom 0: 137.72,134.24 137.94,134.63
S$7393
  Bottom 0: 137.94,134.63 138.06,135.06
S$7394
  Bottom 0: 138.06,135.06 138.11,135.51
S$7395
  Bottom 0: 138.11,135.51 138.06,135.96
S$7396
  Bottom 0: 138.06,135.96 137.94,136.38
S$7397
  Bottom 0: 137.94,136.38 137.72,136.78
S$7398
  Bottom 0: 137.72,136.78 137.44,137.12
S$7399
  Bottom 0: 137.44,137.12 137.09,137.41
S$7400
  Bottom 0: 137.09,137.41 136.69,137.62
S$7401
  Bottom 0: 136.69,137.62 136.27,137.75
S$7402
  Bottom 0: 136.27,137.75 135.82,137.79
S$7403
  Bottom 0: 135.82,137.79 135.38,137.75
S$7404
  Bottom 0: 135.38,137.75 134.95,137.62
S$7405
  Bottom 0: 134.95,137.62 134.55,137.41
S$7406
  Bottom 0: 134.55,137.41 134.21,137.12
S$7407
  Bottom 0: 134.21,137.12 133.92,136.78
S$7408
  Bottom 0: 133.92,136.78 133.71,136.38
S$7409
  Bottom 0: 133.71,136.38 133.58,135.96
S$7410
  Bottom 0: 133.58,135.96 133.54,135.51
S$7411
  Bottom 0: 133.54,135.51 133.58,135.06
S$7412
  Bottom 0: 133.58,135.06 133.71,134.63
S$7413
  Bottom 0: 133.71,134.63 133.92,134.24
S$7414
  Bottom 0: 133.92,134.24 134.21,133.89
S$7415
  Bottom 0: 134.21,133.89 134.55,133.61
S$7416
  Bottom 0: 134.55,133.61 134.95,133.4
S$7417
  Bottom 0: 134.95,133.4 135.38,133.27
S$7418
  Bottom 0: 135.38,133.27 135.82,133.22
S$7419
  Bottom 0: 121.62,149.97 121.92,150.04
S$7420
  Bottom 0: 121.92,150.04 122.18,150.19
S$7421
  Bottom 0: 122.18,150.19 122.39,150.41
S$7422
  Bottom 0: 122.39,150.41 122.52,150.68
S$7423
  Bottom 0: 122.52,150.68 122.56,150.98
S$7424
  Bottom 0: 122.56,150.98 122.52,151.28
S$7425
  Bottom 0: 122.52,151.28 122.39,151.56
S$7426
  Bottom 0: 122.39,151.56 122.18,151.78
S$7427
  Bottom 0: 122.18,151.78 121.92,151.93
S$7428
  Bottom 0: 121.92,151.93 121.62,151.99
S$7429
  Bottom 0: 121.62,151.99 121.32,151.97
S$7430
  Bottom 0: 121.32,151.97 121.04,151.86
S$7431
  Bottom 0: 121.04,151.86 120.8,151.67
S$7432
  Bottom 0: 120.8,151.67 120.64,151.43
S$7433
  Bottom 0: 120.64,151.43 120.54,151.13
S$7434
  Bottom 0: 120.54,151.13 120.54,150.83
S$7435
  Bottom 0: 120.54,150.83 120.64,150.54
S$7436
  Bottom 0: 120.64,150.54 120.8,150.29
S$7437
  Bottom 0: 120.8,150.29 121.04,150.1
S$7438
  Bottom 0: 121.04,150.1 121.32,149.99
S$7439
  Bottom 0: 121.32,149.99 121.62,149.97
S$7440
  Bottom 0: 131.06,152.27 131.51,152.32
S$7441
  Bottom 0: 131.51,152.32 131.94,152.45
S$7442
  Bottom 0: 131.94,152.45 132.33,152.66
S$7443
  Bottom 0: 132.33,152.66 132.68,152.94
S$7444
  Bottom 0: 132.68,152.94 132.96,153.29
S$7445
  Bottom 0: 132.96,153.29 133.18,153.68
S$7446
  Bottom 0: 133.18,153.68 133.3,154.11
S$7447
  Bottom 0: 133.3,154.11 133.35,154.56
S$7448
  Bottom 0: 133.35,154.56 133.3,155.01
S$7449
  Bottom 0: 133.3,155.01 133.18,155.43
S$7450
  Bottom 0: 133.18,155.43 132.96,155.83
S$7451
  Bottom 0: 132.96,155.83 132.68,156.17
S$7452
  Bottom 0: 132.68,156.17 132.33,156.46
S$7453
  Bottom 0: 132.33,156.46 131.94,156.67
S$7454
  Bottom 0: 131.94,156.67 131.51,156.8
S$7455
  Bottom 0: 131.51,156.8 131.06,156.84
S$7456
  Bottom 0: 131.06,156.84 130.62,156.8
S$7457
  Bottom 0: 130.62,156.8 130.19,156.67
S$7458
  Bottom 0: 130.19,156.67 129.79,156.46
S$7459
  Bottom 0: 129.79,156.46 129.45,156.17
S$7460
  Bottom 0: 129.45,156.17 129.16,155.83
S$7461
  Bottom 0: 129.16,155.83 128.95,155.43
S$7462
  Bottom 0: 128.95,155.43 128.82,155.01
S$7463
  Bottom 0: 128.82,155.01 128.78,154.56
S$7464
  Bottom 0: 128.78,154.56 128.82,154.11
S$7465
  Bottom 0: 128.82,154.11 128.95,153.68
S$7466
  Bottom 0: 128.95,153.68 129.16,153.29
S$7467
  Bottom 0: 129.16,153.29 129.45,152.94
S$7468
  Bottom 0: 129.45,152.94 129.79,152.66
S$7469
  Bottom 0: 129.79,152.66 130.19,152.45
S$7470
  Bottom 0: 130.19,152.45 130.62,152.32
S$7471
  Bottom 0: 130.62,152.32 131.06,152.27
S$7472
  Bottom 0: 112.1,169.03 112.39,169.09
S$7473
  Bottom 0: 112.39,169.09 112.66,169.25
S$7474
  Bottom 0: 112.66,169.25 112.86,169.46
S$7475
  Bottom 0: 112.86,169.46 112.99,169.74
S$7476
  Bottom 0: 112.99,169.74 113.04,170.04
S$7477
  Bottom 0: 113.04,170.04 112.99,170.34
S$7478
  Bottom 0: 112.99,170.34 112.86,170.61
S$7479
  Bottom 0: 112.86,170.61 112.66,170.83
S$7480
  Bottom 0: 112.66,170.83 112.39,170.98
S$7481
  Bottom 0: 112.39,170.98 112.1,171.05
S$7482
  Bottom 0: 112.1,171.05 111.8,171.03
S$7483
  Bottom 0: 111.8,171.03 111.52,170.92
S$7484
  Bottom 0: 111.52,170.92 111.28,170.73
S$7485
  Bottom 0: 111.28,170.73 111.11,170.48
S$7486
  Bottom 0: 111.11,170.48 111.02,170.19
S$7487
  Bottom 0: 111.02,170.19 111.02,169.88
S$7488
  Bottom 0: 111.02,169.88 111.11,169.6
S$7489
  Bottom 0: 111.11,169.6 111.28,169.35
S$7490
  Bottom 0: 111.28,169.35 111.52,169.16
S$7491
  Bottom 0: 111.52,169.16 111.8,169.05
S$7492
  Bottom 0: 111.8,169.05 112.1,169.03
S$7493
  Bottom 0: 102.49,171.32 102.94,171.37
S$7494
  Bottom 0: 102.94,171.37 103.36,171.5
S$7495
  Bottom 0: 103.36,171.5 103.76,171.71
S$7496
  Bottom 0: 103.76,171.71 104.1,171.99
S$7497
  Bottom 0: 104.1,171.99 104.39,172.34
S$7498
  Bottom 0: 104.39,172.34 104.6,172.74
S$7499
  Bottom 0: 104.6,172.74 104.73,173.16
S$7500
  Bottom 0: 104.73,173.16 104.78,173.61
S$7501
  Bottom 0: 104.78,173.61 104.73,174.06
S$7502
  Bottom 0: 104.73,174.06 104.6,174.48
S$7503
  Bottom 0: 104.6,174.48 104.39,174.88
S$7504
  Bottom 0: 104.39,174.88 104.1,175.22
S$7505
  Bottom 0: 104.1,175.22 103.76,175.51
S$7506
  Bottom 0: 103.76,175.51 103.36,175.72
S$7507
  Bottom 0: 103.36,175.72 102.94,175.85
S$7508
  Bottom 0: 102.94,175.85 102.49,175.9
S$7509
  Bottom 0: 102.49,175.9 102.04,175.85
S$7510
  Bottom 0: 102.04,175.85 101.61,175.72
S$7511
  Bottom 0: 101.61,175.72 101.22,175.51
S$7512
  Bottom 0: 101.22,175.51 100.87,175.22
S$7513
  Bottom 0: 100.87,175.22 100.59,174.88
S$7514
  Bottom 0: 100.59,174.88 100.37,174.48
S$7515
  Bottom 0: 100.37,174.48 100.25,174.06
S$7516
  Bottom 0: 100.25,174.06 100.2,173.61
S$7517
  Bottom 0: 100.2,173.61 100.25,173.16
S$7518
  Bottom 0: 100.25,173.16 100.37,172.74
S$7519
  Bottom 0: 100.37,172.74 100.59,172.34
S$7520
  Bottom 0: 100.59,172.34 100.87,171.99
S$7521
  Bottom 0: 100.87,171.99 101.22,171.71
S$7522
  Bottom 0: 101.22,171.71 101.61,171.5
S$7523
  Bottom 0: 101.61,171.5 102.04,171.37
S$7524
  Bottom 0: 102.04,171.37 102.49,171.32
S$7525
  Bottom 0: 112.1,176.65 112.39,176.71
S$7526
  Bottom 0: 112.39,176.71 112.66,176.87
S$7527
  Bottom 0: 112.66,176.87 112.86,177.08
S$7528
  Bottom 0: 112.86,177.08 112.99,177.36
S$7529
  Bottom 0: 112.99,177.36 113.04,177.66
S$7530
  Bottom 0: 113.04,177.66 112.99,177.96
S$7531
  Bottom 0: 112.99,177.96 112.86,178.23
S$7532
  Bottom 0: 112.86,178.23 112.66,178.45
S$7533
  Bottom 0: 112.66,178.45 112.39,178.6
S$7534
  Bottom 0: 112.39,178.6 112.1,178.67
S$7535
  Bottom 0: 112.1,178.67 111.8,178.65
S$7536
  Bottom 0: 111.8,178.65 111.52,178.54
S$7537
  Bottom 0: 111.52,178.54 111.28,178.35
S$7538
  Bottom 0: 111.28,178.35 111.11,178.1
S$7539
  Bottom 0: 111.11,178.1 111.02,177.81
S$7540
  Bottom 0: 111.02,177.81 111.02,177.5
S$7541
  Bottom 0: 111.02,177.5 111.11,177.22
S$7542
  Bottom 0: 111.11,177.22 111.28,176.97
S$7543
  Bottom 0: 111.28,176.97 111.52,176.78
S$7544
  Bottom 0: 111.52,176.78 111.8,176.67
S$7545
  Bottom 0: 111.8,176.67 112.1,176.65
S$7546
  Bottom 0: 290.13,95.37 285.16,100.34
S$7547
  Bottom 0: 285.16,100.34 285.1,100.39
S$7548
  Bottom 0: 285.1,100.39 285.04,100.43
S$7549
  Bottom 0: 285.04,100.43 284.98,100.45
S$7550
  Bottom 0: 284.98,100.45 284.91,100.47
S$7551
  Bottom 0: 284.91,100.47 284.84,100.47
S$7552
  Bottom 0: 284.84,100.47 276.97,100.47
S$7553
  Bottom 0: 276.97,100.47 276.11,101.34
S$7554
  Bottom 0: 276.11,101.34 278.18,101.34
S$7555
  Bottom 0: 278.18,101.34 278.25,101.35
S$7556
  Bottom 0: 278.25,101.35 278.32,101.39
S$7557
  Bottom 0: 278.32,101.39 278.38,101.44
S$7558
  Bottom 0: 278.38,101.44 278.42,101.51
S$7559
  Bottom 0: 278.42,101.51 278.43,101.59
S$7560
  Bottom 0: 278.43,101.59 278.43,101.82
S$7561
  Bottom 0: 278.43,101.82 278.45,101.78
S$7562
  Bottom 0: 278.45,101.78 278.69,101.59
S$7563
  Bottom 0: 278.69,101.59 278.97,101.48
S$7564
  Bottom 0: 278.97,101.48 279.28,101.46
S$7565
  Bottom 0: 279.28,101.46 279.4,101.49
S$7566
  Bottom 0: 279.4,101.49 279.49,101.43
S$7567
  Bottom 0: 279.49,101.43 279.8,101.34
S$7568
  Bottom 0: 279.8,101.34 280.12,101.34
S$7569
  Bottom 0: 280.12,101.34 280.44,101.43
S$7570
  Bottom 0: 280.44,101.43 280.71,101.61
S$7571
  Bottom 0: 280.71,101.61 280.81,101.72
S$7572
  Bottom 0: 280.81,101.72 285.22,101.72
S$7573
  Bottom 0: 285.22,101.72 285.22,100.91
S$7574
  Bottom 0: 285.22,100.91 285.22,100.82
S$7575
  Bottom 0: 285.22,100.82 285.25,100.73
S$7576
  Bottom 0: 285.25,100.73 285.28,100.65
S$7577
  Bottom 0: 285.28,100.65 285.33,100.57
S$7578
  Bottom 0: 285.33,100.57 285.38,100.51
S$7579
  Bottom 0: 285.38,100.51 286.11,99.79
S$7580
  Bottom 0: 286.11,99.79 286.18,99.72
S$7581
  Bottom 0: 286.18,99.72 286.25,99.68
S$7582
  Bottom 0: 286.25,99.68 286.34,99.64
S$7583
  Bottom 0: 286.34,99.64 286.43,99.62
S$7584
  Bottom 0: 286.43,99.62 286.51,99.62
S$7585
  Bottom 0: 286.51,99.62 296.46,99.62
S$7586
  Bottom 0: 296.46,99.62 296.1,99.51
S$7587
  Bottom 0: 296.1,99.51 295.7,99.3
S$7588
  Bottom 0: 295.7,99.3 295.36,99.01
S$7589
  Bottom 0: 295.36,99.01 295.07,98.67
S$7590
  Bottom 0: 295.07,98.67 294.86,98.27
S$7591
  Bottom 0: 294.86,98.27 294.73,97.85
S$7592
  Bottom 0: 294.73,97.85 294.69,97.4
S$7593
  Bottom 0: 294.69,97.4 294.73,96.95
S$7594
  Bottom 0: 294.73,96.95 294.86,96.53
S$7595
  Bottom 0: 294.86,96.53 295.07,96.13
S$7596
  Bottom 0: 295.07,96.13 295.36,95.78
S$7597
  Bottom 0: 295.36,95.78 295.7,95.5
S$7598
  Bottom 0: 295.7,95.5 295.95,95.37
S$7599
  Bottom 0: 295.95,95.37 290.13,95.37
S$7600
  Bottom 0: 275.79,96.6 270.96,101.43
S$7601
  Bottom 0: 270.96,101.43 270.96,104.48
S$7602
  Bottom 0: 270.96,104.48 270.95,104.56
S$7603
  Bottom 0: 270.95,104.56 270.94,104.62
S$7604
  Bottom 0: 270.94,104.62 270.91,104.68
S$7605
  Bottom 0: 270.91,104.68 270.87,104.75
S$7606
  Bottom 0: 270.87,104.75 270.83,104.8
S$7607
  Bottom 0: 270.83,104.8 262.33,113.3
S$7608
  Bottom 0: 262.33,113.3 262.43,113.57
S$7609
  Bottom 0: 262.43,113.57 262.48,113.92
S$7610
  Bottom 0: 262.48,113.92 262.43,114.26
S$7611
  Bottom 0: 262.43,114.26 262.31,114.59
S$7612
  Bottom 0: 262.31,114.59 262.1,114.87
S$7613
  Bottom 0: 262.1,114.87 261.83,115.1
S$7614
  Bottom 0: 261.83,115.1 261.79,115.11
S$7615
  Bottom 0: 261.79,115.11 261.79,123.28
S$7616
  Bottom 0: 261.79,123.28 280.94,142.43
S$7617
  Bottom 0: 280.94,142.43 281.05,142.42
S$7618
  Bottom 0: 281.05,142.42 281.3,142.48
S$7619
  Bottom 0: 281.3,142.48 281.5,142.63
S$7620
  Bottom 0: 281.5,142.63 281.63,142.85
S$7621
  Bottom 0: 281.63,142.85 281.68,143.1
S$7622
  Bottom 0: 281.68,143.1 281.63,143.35
S$7623
  Bottom 0: 281.63,143.35 281.5,143.56
S$7624
  Bottom 0: 281.5,143.56 281.3,143.71
S$7625
  Bottom 0: 281.3,143.71 281.13,143.76
S$7626
  Bottom 0: 281.13,143.76 281.22,143.84
S$7627
  Bottom 0: 281.22,143.84 281.57,143.84
S$7628
  Bottom 0: 281.57,143.84 281.67,143.74
S$7629
  Bottom 0: 281.67,143.74 281.89,143.63
S$7630
  Bottom 0: 281.89,143.63 282.14,143.61
S$7631
  Bottom 0: 282.14,143.61 282.39,143.67
S$7632
  Bottom 0: 282.39,143.67 282.59,143.82
S$7633
  Bottom 0: 282.59,143.82 282.72,144.04
S$7634
  Bottom 0: 282.72,144.04 282.77,144.28
S$7635
  Bottom 0: 282.77,144.28 282.72,144.54
S$7636
  Bottom 0: 282.72,144.54 282.59,144.75
S$7637
  Bottom 0: 282.59,144.75 282.39,144.9
S$7638
  Bottom 0: 282.39,144.9 282.14,144.97
S$7639
  Bottom 0: 282.14,144.97 281.89,144.95
S$7640
  Bottom 0: 281.89,144.95 281.67,144.84
S$7641
  Bottom 0: 281.67,144.84 281.57,144.73
S$7642
  Bottom 0: 281.57,144.73 281.04,144.73
S$7643
  Bottom 0: 281.04,144.73 280.97,144.72
S$7644
  Bottom 0: 280.97,144.72 280.9,144.71
S$7645
  Bottom 0: 280.9,144.71 280.84,144.68
S$7646
  Bottom 0: 280.84,144.68 280.78,144.64
S$7647
  Bottom 0: 280.78,144.64 280.73,144.6
S$7648
  Bottom 0: 280.73,144.6 278.97,142.83
S$7649
  Bottom 0: 278.97,142.83 266.49,142.83
S$7650
  Bottom 0: 266.49,142.83 266.69,142.97
S$7651
  Bottom 0: 266.69,142.97 266.89,143.23
S$7652
  Bottom 0: 266.89,143.23 266.91,143.27
S$7653
  Bottom 0: 266.91,143.27 270.64,143.27
S$7654
  Bottom 0: 270.64,143.27 270.73,143.28
S$7655
  Bottom 0: 270.73,143.28 270.81,143.3
S$7656
  Bottom 0: 270.81,143.3 270.9,143.34
S$7657
  Bottom 0: 270.9,143.34 270.97,143.38
S$7658
  Bottom 0: 270.97,143.38 271.04,143.44
S$7659
  Bottom 0: 271.04,143.44 277.2,149.61
S$7660
  Bottom 0: 277.2,149.61 277.46,149.56
S$7661
  Bottom 0: 277.46,149.56 277.79,149.58
S$7662
  Bottom 0: 277.79,149.58 278.09,149.69
S$7663
  Bottom 0: 278.09,149.69 278.35,149.87
S$7664
  Bottom 0: 278.35,149.87 278.56,150.13
S$7665
  Bottom 0: 278.56,150.13 278.69,150.43
S$7666
  Bottom 0: 278.69,150.43 278.74,150.75
S$7667
  Bottom 0: 278.74,150.75 278.7,150.95
S$7668
  Bottom 0: 278.7,150.95 283.09,146.56
S$7669
  Bottom 0: 283.09,146.56 283.09,142.22
S$7670
  Bottom 0: 283.09,142.22 283.05,142.17
S$7671
  Bottom 0: 283.05,142.17 282.96,141.93
S$7672
  Bottom 0: 282.96,141.93 282.96,141.86
S$7673
  Bottom 0: 282.96,141.86 270.9,129.8
S$7674
  Bottom 0: 270.9,129.8 270.85,129.75
S$7675
  Bottom 0: 270.85,129.75 270.81,129.69
S$7676
  Bottom 0: 270.81,129.69 270.79,129.63
S$7677
  Bottom 0: 270.79,129.63 270.77,129.56
S$7678
  Bottom 0: 270.77,129.56 270.77,129.49
S$7679
  Bottom 0: 270.77,129.49 270.77,128.06
S$7680
  Bottom 0: 270.77,128.06 268.4,128.06
S$7681
  Bottom 0: 268.4,128.06 268.39,128.08
S$7682
  Bottom 0: 268.39,128.08 268.19,128.23
S$7683
  Bottom 0: 268.19,128.23 267.94,128.29
S$7684
  Bottom 0: 267.94,128.29 267.7,128.28
S$7685
  Bottom 0: 267.7,128.28 267.47,128.16
S$7686
  Bottom 0: 267.47,128.16 267.3,127.97
S$7687
  Bottom 0: 267.3,127.97 267.21,127.74
S$7688
  Bottom 0: 267.21,127.74 267.21,127.49
S$7689
  Bottom 0: 267.21,127.49 267.3,127.25
S$7690
  Bottom 0: 267.3,127.25 267.47,127.07
S$7691
  Bottom 0: 267.47,127.07 267.7,126.95
S$7692
  Bottom 0: 267.7,126.95 267.94,126.93
S$7693
  Bottom 0: 267.94,126.93 268.19,127
S$7694
  Bottom 0: 268.19,127 268.39,127.15
S$7695
  Bottom 0: 268.39,127.15 268.4,127.17
S$7696
  Bottom 0: 268.4,127.17 270.77,127.17
S$7697
  Bottom 0: 270.77,127.17 270.77,105.6
S$7698
  Bottom 0: 270.77,105.6 270.77,105.53
S$7699
  Bottom 0: 270.77,105.53 270.79,105.47
S$7700
  Bottom 0: 270.79,105.47 270.81,105.41
S$7701
  Bottom 0: 270.81,105.41 270.85,105.34
S$7702
  Bottom 0: 270.85,105.34 270.9,105.29
S$7703
  Bottom 0: 270.9,105.29 276.47,99.72
S$7704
